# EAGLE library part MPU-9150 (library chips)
GYRO/ACCELEROMETER 9-AXIS 24LGA
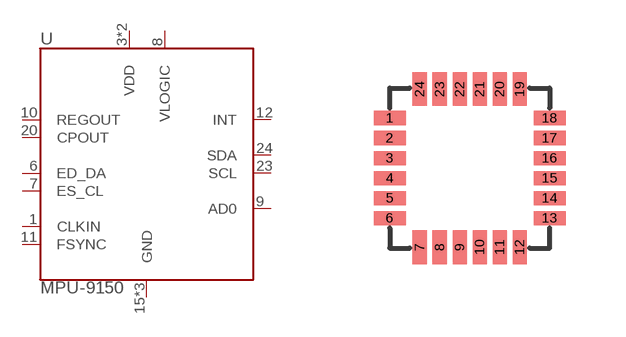
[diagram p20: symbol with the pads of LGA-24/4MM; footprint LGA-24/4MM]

Designator prefix U

## MPU-9150 (DIGIKEY: 1428-1009-1-ND)  [LGA-24/4MM]
1  CLKIN
3  VDD
6  ED_DA
7  ES_CL
8  VLOGIC
9  AD0
10  REGOUT
11  FSYNC
12  INT
13  VDD
15  GND
17  GND
18  GND
20  CPOUT
23  SCL
24  SDA

## Footprint LGA-24/4MM (pad centres in mm)
smd 0.8 x 0.35: 1 -2,1.25; 2 -2,0.75; 3 -2,0.25; 4 -2,-0.25; 5 -2,-0.75; 6 -2,-1.25; 13 2,-1.25; 14 2,-0.75; 15 2,-0.25; 16 2,0.25; 17 2,0.75; 18 2,1.25
smd 0.35 x 0.85: 7 -1.25,-1.975; 8 -0.75,-1.975; 9 -0.25,-1.975; 10 0.25,-1.975; 11 0.75,-1.975; 12 1.25,-1.975; 19 1.25,1.975; 20 0.75,1.975; 21 0.25,1.975; 22 -0.25,1.975; 23 -0.75,1.975; 24 -1.25,1.975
